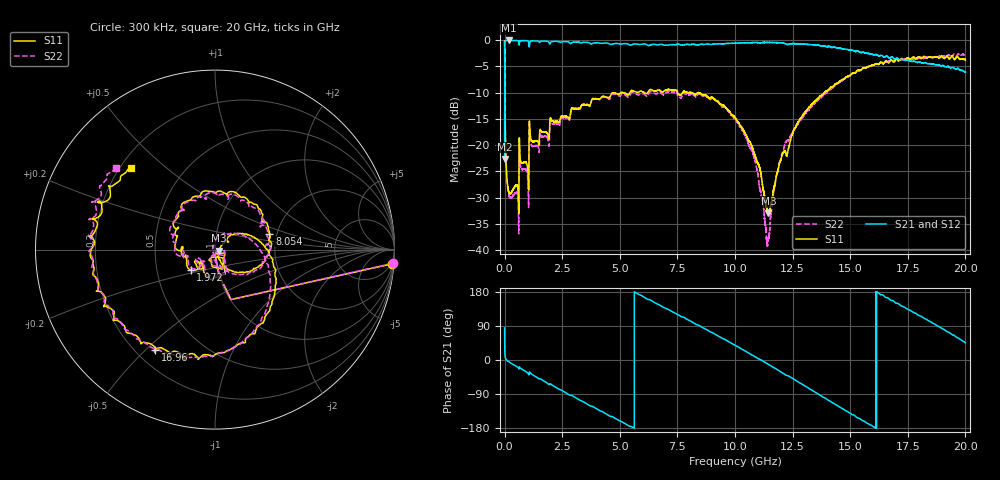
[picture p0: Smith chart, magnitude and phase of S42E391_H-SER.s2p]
! Created Wed Nov 25 22:15:28 2020
# khz S ma R 50
! 2 Port Network Data from SP1.SP block
! freq  magS11  angS11  magS21  angS21  magS12  angS12  magS22  angS22
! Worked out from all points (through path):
!   20001 points, 300 kHz to 20 GHz, reference 50 ohm
!   highest |S21| = -0.06 dB at 192.3 MHz (marker M1); lowest = -22.7 dB at 300 kHz (marker M2)
!   group delay of S21, straight-line fit = 93.7 ps
!   lowest |S11| = -33.0 dB at 11.45 GHz (marker M3), VSWR 1.05, Z = 52.2 - j0.572 ohm
!   |S11| at or under -10 dB: 12.19 MHz to 5.055 GHz (5.042 GHz wide, 199 % of centre); 5.136 GHz to 5.436 GHz (300.5 MHz wide, 5.68 % of centre); 8.425 GHz to 13.89 GHz (5.46 GHz wide, 48.9 % of centre)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
!   |S22| runs from -39.3 to -0.1 dB; largest |S21 - S12| = 0.015
!   S11 on the Smith chart (normalised r, x): 300 kHz: 3, -25; 1.972 GHz: 0.75, -0.18; 8.054 GHz: 1.83, +0.36; 16.96 GHz: 0.28, -0.53; 20 GHz: 0.25, +0.39
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300  0.9901 -4.6  0.07356 84.7  0.07316 84.6  0.9923 -4.5
101300  0.04758 -83.8  0.9915 -1.1  0.9923 -1.1  0.04654 -83.5
192300  0.03541 -86.2  0.9935 -5.2  0.9917 -5.2  0.03309 -86.0
522300  0.04176 -99.7  0.9911 -17.2  0.9916 -17.2  0.03517 -99.9
724300  0.06775 -109.9  0.9893 -23.3  0.9895 -23.3  0.05946 -110.4
955300  0.06716 -119.4  0.9889 -31.9  0.9876 -31.8  0.05697 -121.0
1158300  0.112 -126.5  0.9816 -36.7  0.9823 -36.8  0.1008 -125.8
1972300  0.1768 -139.5  0.9256 -62.9  0.9256 -63.0  0.1625 -138.7
3334300  0.2379 158.6  0.9432 -107.7  0.9436 -107.7  0.2364 169.4
5202300  0.3119 107.6  0.9258 -167.0  0.9247 -167.0  0.3033 103.6
6667300  0.3352 59.4  0.9033 147.1  0.9025 147.0  0.3179 59.8
8054300  0.3161 16.3  0.9054 103.3  0.9052 103.3  0.3023 13.1
1.00003e7  0.184 -44.6  0.9355 39.1  0.9349 39.1  0.1799 -49.9
1.08133e7  0.08559 -65.1  0.9492 10.9  0.9502 10.9  0.07848 -82.2
1.14533e7  0.02232 -14.2  0.9525 -11.6  0.9524 -11.6  0.01288 155.2
1.21273e7  0.08669 31.7  0.9351 -36.7  0.934 -36.7  0.09419 63.2
1.33343e7  0.2432 13.0  0.9044 -79.6  0.9045 -79.6  0.2345 5.5
1.50303e7  0.4685 -53.6  0.8004 -142.1  0.8022 -142.0  0.4654 -56.1
1.66673e7  0.6083 -109.6  0.6806 162.8  0.6834 162.0  0.6277 -108.1
1.69613e7  0.6496 -120.8  0.6645 151.3  0.6738 151.7  0.64 -117.1
1.87003e7  0.6953 -177.5  0.5818 93.3  0.5872 93.3  0.6825 -174.3
2e7  0.6492 135.6  0.4959 45.5  0.4958 45.9  0.7233 140.2
